(* Logix 5000 AddOnInstructionDefinition export CM1T_CMLWriteRegister; software revision 20.00 *)

TYPE CM1T_CMLDriveStatus :
STRUCT
   StatusValue : SINT;   // Indicates status and error type
   StatusValue1 : SINT;   // Additional status values
   In_Position : BOOL;   // Drive is in position and ready to move
   Moving : BOOL;   // Drive is currently moving
   Disabled : BOOL;   // Drive is disabled
   Error : BOOL;   // Drive is in an error state
   HomeAchieved : BOOL;   // Home achieved
END_STRUCT
END_TYPE

TYPE CM1T_CMLAxis :   // CML Axis
STRUCT
   Input : SINT[60];   // Data coming from the CM1-T
   Output : SINT[44];   // Data going to the CM1-T
   us50Counter : DINT;   // Controller 50us counter
   DriveStatus : CM1T_CMLDriveStatus;   // Shows status of the drive
   PositionActual : DINT;   // Actual position of the drive
   TargetActual : DINT;   // 1ms position target
   PositionError : DINT;   // Error between the current drive position and the instantaneous target position
   SpeedActual : DINT;   // Actual speed of the drive
   CurrentActual : INT;   // 0.1% of rated current
   OverloadActual : INT;   // 0.1% of overload torque
   DCVoltage : INT;   // DC voltage bus. 0.1V unit
   AnalogIN : INT;   // Value of 10bit analog input
   DigitalIN : SINT;   // Read the digital inputs
   DigitalOUT : SINT;   // Set the digital outputs
   Temperature : SINT;   // Temperature of the drive
   ErrorCode : SINT;   // Indicates error in Ethernet/IP module
   WriteValue : DINT[5];   // Write value array
   ReadValue : DINT[5];   // Read Value array
   WriteAddr : INT[5];   // Write Address array
   ReadAddr : INT[5];   // Read Address array
   ReadValueAddr : INT[5];   // Address of ReadValue
END_STRUCT
END_TYPE

ADD_ON_INSTRUCTION CM1T_CMLWriteRegister   (* revision 1.0 *)
// WriteRegister
VAR_IN_OUT
   CM1T_CMLAxis : CM1T_CMLAxis; {required}
END_VAR
VAR_INPUT
   Slot : SINT; {required}
   Address : INT; {required}
   Value : DINT; {access Read Only, required}
END_VAR
VAR_OUTPUT
   Done : BOOL; {access Read Only, visible}
END_VAR
VAR
   usCount : DINT; {access None}
END_VAR

ROUTINE Logic   (* ladder *)
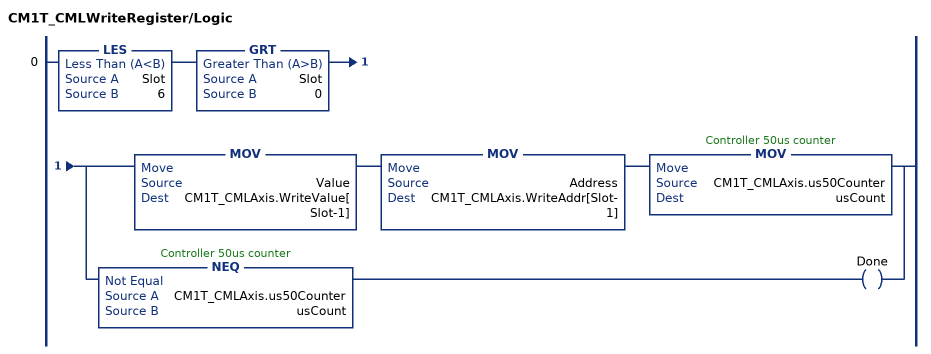
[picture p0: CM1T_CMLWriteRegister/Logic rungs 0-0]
   0: LES(Slot,6)GRT(Slot,0)[MOV(Value,CM1T_CMLAxis.WriteValue[Slot-1]) MOV(Address,CM1T_CMLAxis.WriteAddr[Slot-1]) MOV(CM1T_CMLAxis.us50Counter,usCount) ,NEQ(CM1T_CMLAxis.us50Counter,usCount) OTE(Done) ];
END_ROUTINE
END_ADD_ON_INSTRUCTION
